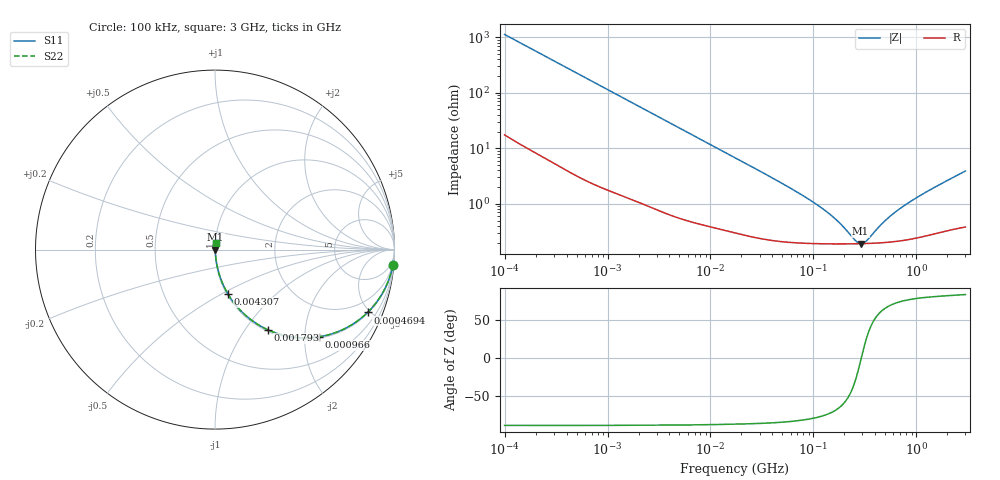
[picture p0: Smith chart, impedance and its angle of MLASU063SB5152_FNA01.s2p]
! MLASU063SB5152_FNA01  S-PARAMETER MODEL  ( Standard Model )
! Model Generated by TAIYO YUDEN Corporation (http://www.ty-top.com)
! Version 1.0
! TAIYO YUDEN Control No. 220601
! Copyright(c) 2013 TAIYO YUDEN CO.,LTD. All Rights Reserved.
! Product Description (link to TY-COMPAS)
! https://ds.yuden.co.jp/TYCOMPAS/or/detail?pn=MLASU063SB5152KFNA01&u=M
! Products Name : Multilayer Ceramic Capacitors
! Characteristics :
!  Capacitance : 1500 [pF] , Rated Voltage : 50 [V] , TCC : B / X5R
!  Case Size : 0.6 x 0.3 / 0.024 x 0.012 [mm/inch] , Thickness : 0.3 / 0.012 [mm/inch]
!  (Conditions: Temperature = 25 [degC] , DC Bias Voltage = 0 [V])
! External Node Assignments :
!  1  o---| |---o  2
! GND o---------o GND
! Frequency Range : 100kHz  -  3GHz  [ 401 STEP ]
# MHZ S RI R 50
! Freq[MHz].  S11 Real  S11 Imag  S21 Real  S21 Imag  S12 Real  S12 Imag  S22 Real  S22 Imag
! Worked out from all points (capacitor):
!   401 points, 100 kHz to 3 GHz, reference 50 ohm
!   read as one part in series: C = 1.42 nF near 105.3 kHz
!   lowest |Z| = 192 mohm at 287.5 MHz (marker M1)
!   series resonance near 291.9 MHz, so ESL is about 210 pH
!   S11 on the Smith chart (normalised r, x): 100 kHz: 1, -22; 469.4 kHz: 1.07, -4.83; 966 kHz: 1.04, -2.36; 1.793 MHz: 1.02, -1.28; 4.307 MHz: 1.01, -0.54; 3 GHz: 1.01, +0.08
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0.1  0.9907 -0.0883  0.00926 0.0883  0.00926 0.0883  0.9907 -0.0883
0.252895  0.9494 -0.2121  0.0506 0.2121  0.0506 0.2121  0.9494 -0.2121
0.469427  0.8502 -0.3499  0.1498 0.3499  0.1498 0.3499  0.8502 -0.3499
0.562235  0.7997 -0.3933  0.2003 0.3933  0.2003 0.3933  0.7997 -0.3933
0.965977  0.5807 -0.4858  0.4193 0.4858  0.4193 0.4858  0.5807 -0.4858
1.316074  0.431 -0.4869  0.569 0.4869  0.569 0.4869  0.431 -0.4869
1.793056  0.2935 -0.4464  0.7065 0.4464  0.7065 0.4464  0.2935 -0.4464
3.161081  0.1224 -0.3177  0.8776 0.3177  0.8776 0.3177  0.1224 -0.3177
4.306746  0.0721 -0.2476  0.9279 0.2476  0.9279 0.2476  0.0721 -0.2476
8.417093  0.0227 -0.1345  0.9773 0.1345  0.9773 0.1345  0.0227 -0.1345
17.7727  0.00724 -0.0653  0.9928 0.0653  0.9928 0.0653  0.00724 -0.0653
51.12795  0.00257 -0.0224  0.9974 0.0224  0.9974 0.0224  0.00257 -0.0224
97.38194  0.00204 -0.0108  0.998 0.0108  0.998 0.0108  0.00204 -0.0108
154.8634  0.00192 -0.00551  0.9981 0.00551  0.9981 0.00551  0.00192 -0.00551
190.323  0.00191 -0.00358  0.9981 0.00358  0.9981 0.00358  0.00191 -0.00358
252.704  0.0019 -0.00118  0.9981 0.00118  0.9981 0.00118  0.0019 -0.00118
287.4592  0.00191 -0.000125  0.9981 0.000125  0.9981 0.000125  0.00191 -0.000125
326.9943  0.00193 0.000924  0.9981 -0.000924  0.9981 -0.000924  0.00193 0.000924
547.5153  0.00207 0.00543  0.9979 -0.00543  0.9979 -0.00543  0.00207 0.00543
726.971  0.00224 0.00842  0.9978 -0.00842  0.9978 -0.00842  0.00224 0.00842
1042.837  0.00262 0.0131  0.9974 -0.0131  0.9974 -0.0131  0.00262 0.0131
3000  0.0053 0.0385  0.9947 -0.0385  0.9947 -0.0385  0.0053 0.0385
